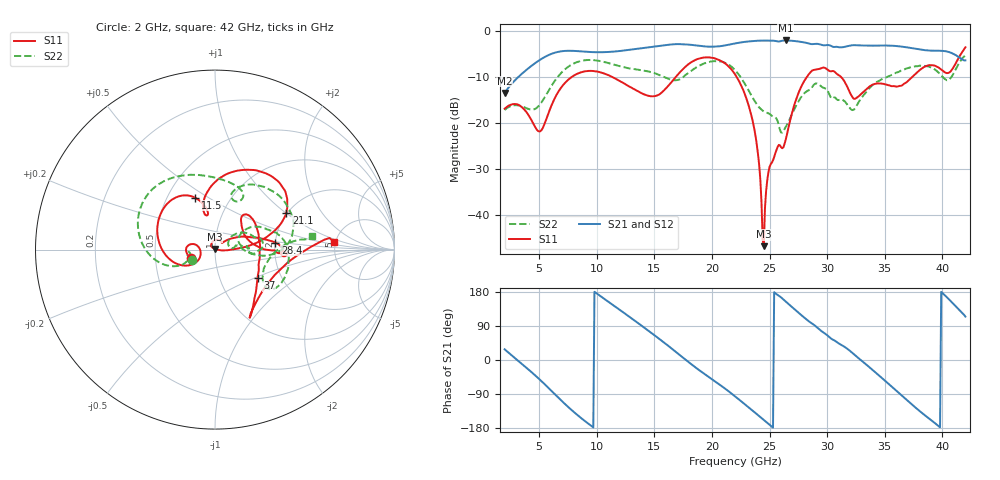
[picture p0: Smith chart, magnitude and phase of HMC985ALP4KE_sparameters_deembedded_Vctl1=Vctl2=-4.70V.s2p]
!s2p File: Measurements: S11, S21, S12, S22
# GHz S dB R 50.0
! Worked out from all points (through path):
!   401 points, 2 GHz to 42 GHz, reference 50 ohm
!   highest |S21| = -2.06 dB at 26.4 GHz (marker M1); lowest = -13.4 dB at 2 GHz (marker M2)
!   lowest |S11| = -46.7 dB at 24.5 GHz (marker M3), VSWR 1.01, Z = 49.8 + j0.423 ohm
!   |S11| at or under -10 dB: start of sweep to 7.816 GHz; 22.15 GHz to 28.23 GHz (6.081 GHz wide, 24.1 % of centre); 31.21 GHz to 37.38 GHz (6.164 GHz wide, 18 % of centre)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
!   |S22| runs from -22.0 to -5.3 dB; largest |S21 - S12| = 0.00076
!   S11 on the Smith chart (normalised r, x): 2 GHz: 0.76, -0.07; 11.5 GHz: 0.69, +0.44; 21.1 GHz: 1.97, +1.02; 28.4 GHz: 2.00, +0.18; 37 GHz: 1.51, -0.52; 42 GHz: 4.85, +0.76
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2  -16.86 -161.8  -13.44 28.2  -13.44 28.2  -17.15 -155.6
5  -21.80 -172.8  -6.38 -50.2  -6.38 -50.2  -16.15 -159.9
6.3  -14.86 -150.4  -4.76 -88.4  -4.76 -88.4  -11.02 -161.7
8.7  -8.92 150.3  -4.44 -154.6  -4.44 -154.6  -6.46 151.2
11.5  -10.18 111.0  -4.47 143.1  -4.47 143.1  -7.31 105.0
13.6  -13.13 101.2  -3.85 97.1  -3.85 97.1  -8.41 75.5
15.4  -13.80 106.0  -3.25 56.3  -3.25 56.3  -9.52 62.0
17.9  -7.31 80.1  -2.94 -3.7  -2.94 -3.7  -9.19 72.0
21.1  -6.98 27.5  -3.15 -74.6  -3.15 -74.6  -6.87 15.9
22  -9.38 16.9  -2.71 -95.8  -2.71 -95.8  -8.47 0.4
23.6  -20.32 0.3  -2.18 -135.5  -2.18 -135.5  -14.77 -4.4
24.5  -46.67 113.7  -2.08 -158.2  -2.08 -158.1  -17.42 8.3
25  -29.48 131.3  -2.10 -170.9  -2.10 -170.9  -17.99 11.1
26.4  -23.59 41.5  -2.06 154.4  -2.06 154.4  -20.87 33.0
28.4  -9.41 6.7  -2.72 102.4  -2.72 102.4  -12.86 18.1
28.7  -8.59 1.8  -2.85 96.2  -2.86 96.2  -12.18 16.2
30.7  -8.98 -3.2  -3.45 50.3  -3.45 50.3  -14.45 2.0
32.5  -14.60 32.1  -3.10 10.5  -3.09 10.5  -16.46 27.8
35.4  -11.80 19.0  -3.17 -65.0  -3.17 -65.0  -9.78 19.3
37  -10.88 -33.9  -3.59 -108.1  -3.59 -108.1  -8.06 4.8
39.8  -8.16 -57.3  -4.29 -177.8  -4.29 -177.7  -9.34 -35.8
42  -3.54 3.8  -6.38 114.5  -6.38 114.5  -5.29 8.2
